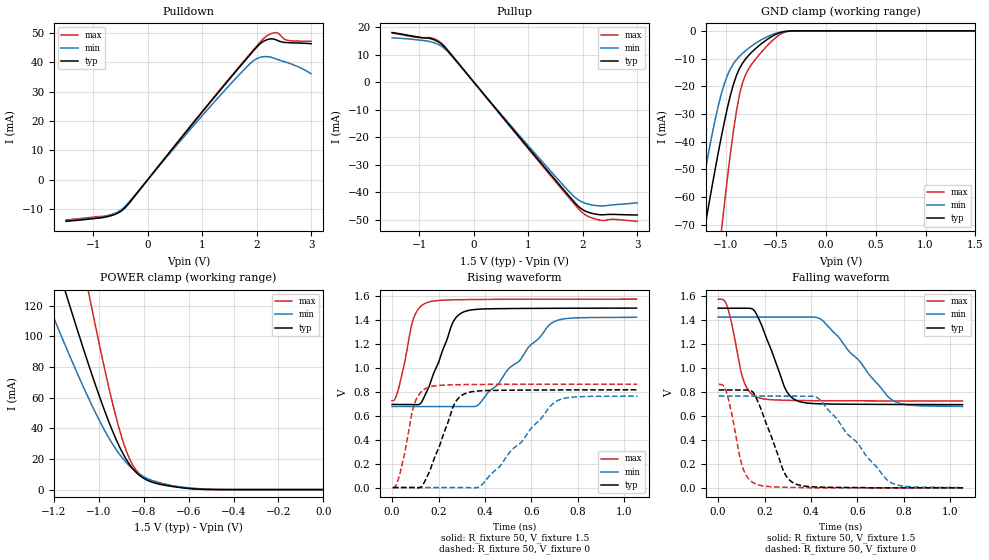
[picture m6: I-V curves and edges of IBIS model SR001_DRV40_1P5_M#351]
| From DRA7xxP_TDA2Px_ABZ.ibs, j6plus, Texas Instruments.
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| Model based on original model for DDR_SEIOPB_H
|   Sub model SR001_DRV40_1P5
[model]   SR001_DRV40_1P5_M#351
|[Description]  [1.5V-I/O-X-X]
|   , ,
|[Input Load]
|[Output Drive]
|Voltage   1.5V
|Mode   I/O
Model_type   I/O
Polarity   Non-Inverting
Enable   Active-Low
Vinl =  0.65
Vinh =  0.85
Cref =  15.0000pF
Rref =  100.0000M
Vref =  0V
Vmeas =  0.75
C_comp   2p   2p   2p
[Model Spec]
Vinl   0.65   0.6125   0.6875
Vinh   0.85   0.8125   0.8875
[Receiver Thresholds]
Tslew_ac = 0.5n
Vth = 0.75
Vth_max = 0.7875
Vth_min = 0.675
Vinh_ac = 0.175
Vinh_dc = 0.1
Vinl_ac = -0.175
Vinl_dc = -0.1
[Temperature Range]   25   125   -40
[Voltage Range]   1.5   1.425   1.575
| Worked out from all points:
|   slope of the pulldown table from 0 to 0.225 V, typ, clamps not added: 43 ohm
|   slope of the pullup table from 0 to 0.225 V, typ, clamps not added: 41.7 ohm
|   GND clamp passes 1 mA (typ) near -0.48 V on its own axis
|   POWER clamp passes 1 mA (typ) near -0.62 V on its own axis
|   rising waveform, R_fixture 50, V_fixture 1.5: 20-80 % time 91.4ps typ, 211ps min, 54.4ps max; typ from 0.695 V to 1.5 V
|   rising waveform, R_fixture 50, V_fixture 0: 20-80 % time 91.4ps typ, 205ps min, 54.2ps max; typ from 0 V to 0.817 V
|   falling waveform, R_fixture 50, V_fixture 1.5: 20-80 % time 91.7ps typ, 194ps min, 55.4ps max; typ from 1.5 V to 0.695 V
|   falling waveform, R_fixture 50, V_fixture 0: 20-80 % time 91.7ps typ, 198ps min, 55.1ps max; typ from 0.817 V to 0 V
[POWER_clamp]
-1.5V     302.8mA    223.9mA    484.4mA
-1.242V   174.3mA    127.3mA    279.1mA
-1.136V   123.3mA    89.68mA    196.8mA
-1.045V   81.65mA    59.62mA    128.8mA
-1.03V    75mA       54.92mA    117.8mA
-939.4mV  38.44mA    29.91mA    56.84mA
-893.9mV  23.93mA    20.41mA    32.31mA
-848.5mV  13.61mA    13.43mA    15.91mA
-803mV    7.623mA    8.663mA    8.564mA
-712.1mV  3.022mA    3.561mA    3.877mA
-575.8mV  470.5uA    872uA      449uA
0V        112.6nA    435.6nA    613.8nA
[Pulldown]
-1.5V     -14.18mA   -14.05mA   -13.7mA
-727.3mV  -12.54mA   -12.27mA   -12.15mA
-545.5mV  -11.35mA   -10.95mA   -11.1mA
-409.1mV  -9.378mA   -8.925mA   -9.416mA
1.227V    28.16mA    26.58mA    28.43mA
1.818V    41.23mA    38.42mA    41.56mA
2V        45.11mA    41.2mA     45.49mA
2.182V    47.62mA    41.92mA    48.94mA
2.273V    47.99mA    41.65mA    49.78mA
2.364V    47.57mA    41.06mA    50.1mA
2.545V    46.7mA     39.96mA    47.58mA
3V        46.28mA    36.09mA    47.12mA
[Pullup]
-1.5V     17.97mA    16.01mA    17.82mA
-1V       16.28mA    15.23mA    16.1mA
-772.7mV  15.66mA    14.54mA    16.02mA
-590.9mV  13.75mA    12.97mA    14.08mA
-409.1mV  9.799mA    9.534mA    9.955mA
1.409V    -33.42mA   -32.26mA   -33.94mA
1.773V    -41.87mA   -40.19mA   -42.52mA
1.909V    -44.87mA   -42.6mA    -45.68mA
2.091V    -47.15mA   -44.23mA   -48.65mA
2.318V    -48.13mA   -44.93mA   -50.11mA
2.591V    -48.02mA   -44.49mA   -49.82mA
3V        -48.22mA   -43.8mA    -50.51mA
[GND_clamp]
-1.5V     -133.6mA   -115.7mA   -234.3mA
-1.288V   -87.29mA   -67.59mA   -156.8mA
-1.197V   -68.11mA   -48.64mA   -124.4mA
-1.045V   -38.25mA   -22.77mA   -72.51mA
-1.015V   -32.88mA   -19.1mA    -62.74mA
-954.5mV  -23.3mA    -13.72mA   -44.4mA
-863.6mV  -13.6mA    -9.192mA   -23.11mA
-803mV    -10.18mA   -7.193mA   -15.89mA
-681.8mV  -5.771mA   -4.027mA   -9.287mA
-500mV    -1.264mA   -914.7uA   -2.429mA
-348.5mV  -52.39uA   -75.11uA   -85.87uA
1.5V      112.6nA    528.1nA    514.5nA
[Ramp]
dV/dt_f 0.48363761/91.775383p 0.44915872/0.19425367n 0.50998988/55.400702p
dV/dt_r   0.49185/91.735492p 0.46127553/0.20596048n 0.52007823/54.40581p
R_load = 50
[Rising Waveform]
R_fixture = 50
V_fixture = 1.5
V_fixture_min = 1.425
V_fixture_max = 1.575
0s        694.7mV    677.7mV    726.2mV
28.68ps   694mV      677.6mV    832mV
91.57ps   693.5mV    677.6mV    1.409V
121.8ps   701.4mV    677.6mV    1.512V
145.3ps   787.4mV    677.6mV    1.542V
260ps     1.372V     677.5mV    1.569V
308.5ps   1.468V     676.7mV    1.571V
374.1ps   1.491V     695.7mV    1.572V
695.2ps   1.498V     1.384V     1.575V
1.053ns   1.5V       1.425V     1.575V
[Rising Waveform]
R_fixture = 50
V_fixture = 0
V_fixture_min = 0
V_fixture_max = 0
3.003ps   0V         0V         0V
32.14ps   0V         0V         105.4mV
95.86ps   0V         0V         697.2mV
122.7ps   0V         0V         794.5mV
148.8ps   83.82mV    0V         831.6mV
265ps     684.6mV    0V         859.1mV
313.6ps   784.7mV    0V         860.7mV
385.9ps   809.1mV    21.05mV    862mV
710.4ps   815.8mV    724.1mV    863.8mV
1.056ns   817.1mV    766.1mV    864.1mV
[Falling Waveform]
R_fixture = 50
V_fixture = 1.5
V_fixture_min = 1.425
V_fixture_max = 1.575
0s        1.5V       1.425V     1.575V
25.58ps   1.5V       1.425V     1.565V
40.91ps   1.5V       1.425V     1.504V
113.5ps   1.5V       1.425V     875.9mV
167.6ps   1.441V     1.425V     756.8mV
288.2ps   831.3mV    1.425V     731.1mV
339.1ps   728.1mV    1.425V     729.4mV
449.4ps   700.8mV    1.397V     727.3mV
756.4ps   696.1mV    725.4mV    725.7mV
1.053ns   694.7mV    677.7mV    725.4mV
[Falling Waveform]
R_fixture = 50
V_fixture = 0
V_fixture_min = 0
V_fixture_max = 0
3.003ps   817.1mV    766.1mV    864.1mV
23.57ps   817.3mV    766.1mV    851.1mV
38.35ps   817.3mV    766.1mV    783.4mV
107ps     816.9mV    766.2mV    163.1mV
160.3ps   765.9mV    766.2mV    33.55mV
283.6ps   132.7mV    766.1mV    5.18mV
332.6ps   33.54mV    765.9mV    3.358mV
436.4ps   6.368mV    739.6mV    0V
744.7ps   0V         44.16mV    0V
1.056ns   0V         0V         0V
